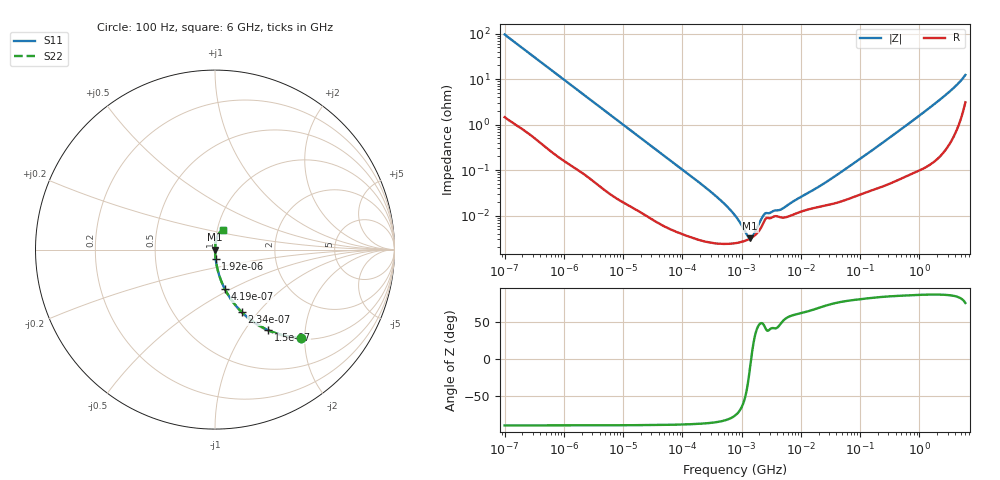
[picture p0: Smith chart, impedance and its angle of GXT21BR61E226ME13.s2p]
!Murata Part Number: GXT21BR61E226ME13
!These Parameters are Measured in Series Mode Connection
!Data Generated on Jan 08, 2026
!  o--ll--o
!Port1  Port2
!  o------o
!Operation Temp=25[degC], DC Bias Voltage=0[V]
!Freq. Start=100[Hz] Stop=6[GHz] 401[Steps]
# Hz S RI R 50
!Freq.(Hz) S11(Real) S11(Imag) S21(Real) S21(Imag) S12(Real) S12(Imag) S22(Real) S22(Imag)
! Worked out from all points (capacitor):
!   401 points, 100 Hz to 6 GHz, reference 50 ohm
!   read as one part in series: C = 16.5 uF near 109 Hz
!   lowest |Z| = 3.18 mohm at 1.386 MHz (marker M1)
!   S11 on the Smith chart (normalised r, x): 100 Hz: 1.03, -1.92; 150 Hz: 1.02, -1.29; 234 Hz: 1.01, -0.83; 419 Hz: 1.01, -0.47; 1.92 kHz: 1.00, -0.10; 6 GHz: 1.06, +0.24
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100  0.4797 -0.4921  0.5203 0.4921  0.5203 0.4921  0.4797 -0.4921
150  0.2959 -0.4486  0.7041 0.4486  0.7041 0.4486  0.2959 -0.4486
234  0.15 -0.3489  0.85 0.3489  0.85 0.3489  0.15 -0.3489
419  0.0545 -0.219  0.9455 0.219  0.9455 0.219  0.0545 -0.219
820  0.0159 -0.1174  0.9841 0.1174  0.9841 0.1174  0.0159 -0.1174
1920  0.00355 -0.0513  0.9964 0.0513  0.9964 0.0513  0.00355 -0.0513
2008  0.00329 -0.0491  0.9967 0.0491  0.9967 0.0491  0.00329 -0.0491
6433  0.000521 -0.0156  0.9995 0.0156  0.9995 0.0156  0.000521 -0.0156
40335  7.33e-05 -0.00254  0.9999 0.00254  0.9999 0.00254  7.33e-05 -0.00254
302498  2.53e-05 -0.000332  1 0.000332  1 0.000332  2.53e-05 -0.000332
495019  2.38e-05 -0.000188  1 0.000188  1 0.000188  2.38e-05 -0.000188
774597  2.46e-05 -9.76e-05  1 9.76e-05  1 9.76e-05  2.46e-05 -9.76e-05
847162  2.5e-05 -8.24e-05  1 8.24e-05  1 8.24e-05  2.5e-05 -8.24e-05
1386327  3.11e-05 -6.6e-06  1 6.6e-06  1 6.6e-06  3.11e-05 -6.6e-06
2169299  5.63e-05 6.37e-05  0.9999 -6.37e-05  0.9999 -6.37e-05  5.63e-05 6.37e-05
4643984  9.07e-05 0.000102  0.9999 -0.000102  0.9999 -0.000102  9.07e-05 0.000102
1.555665e7  0.000143 0.000323  0.9999 -0.000323  0.9999 -0.000323  0.000143 0.000323
3.983537e7  0.00019 0.000744  0.9998 -0.000744  0.9998 -0.000744  0.00019 0.000744
3.124326e8  0.000524 0.00509  0.9995 -0.00509  0.9995 -0.00509  0.000524 0.00509
2.34314e9  0.0035 0.037  0.9965 -0.037  0.9965 -0.037  0.0035 0.037
3.8344e9  0.00958 0.0634  0.9904 -0.0634  0.9904 -0.0634  0.00958 0.0634
6e9  0.043 0.1112  0.957 -0.1112  0.957 -0.1112  0.043 0.1112
